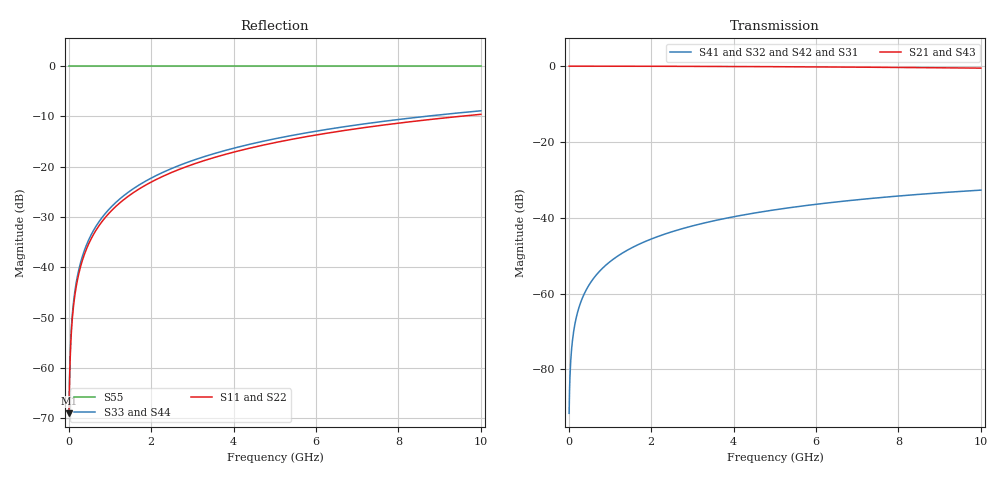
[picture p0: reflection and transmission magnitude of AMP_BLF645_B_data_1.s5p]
! Created Mon Mar  8 11:09:34 2010
# ghz S ma R 50
! 5 Port Network Data from SP1.SP block
! freq  magS11  angS11  magS12  angS12  magS13  angS13  magS14  angS14
!  magS15  angS15
!  magS21  angS21  magS22  angS22  magS23  angS23
!  magS24  angS24  magS25  angS25
!  magS31  angS31  magS32  angS32
!  magS33  angS33  magS34  angS34  magS35  angS35
!  magS41  angS41
!  magS42  angS42  magS43  angS43  magS44  angS44  magS45  angS45
!  magS51  angS51  magS52  angS52  magS53  angS53  magS54  angS54
!  magS55  angS55
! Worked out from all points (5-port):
!   1000 points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, 10 MHz to 10 GHz, reference 50 ohm
!   strongest paths, dB at 10 MHz, 2.51 GHz, 5.01 GHz, 7.51 GHz, 10 GHz:
!     S21: 0.0, 0.0, -0.1, -0.3, -0.5
!     S43: 0.0, 0.0, -0.2, -0.4, -0.6
!     S41: -91.6, -43.7, -37.9, -34.7, -32.7
!     S32: -91.6, -43.7, -37.9, -34.7, -32.7
!     S42: -91.6, -43.7, -37.9, -34.7, -32.7
!     S31: -91.6, -43.7, -37.9, -34.7, -32.7
!   lowest |S11| = -69.1 dB at 10 MHz (marker M1), VSWR 1.00, Z = 50 + j0.0352 ohm
!   |S11| at or under -10 dB: start of sweep to 9.472 GHz
